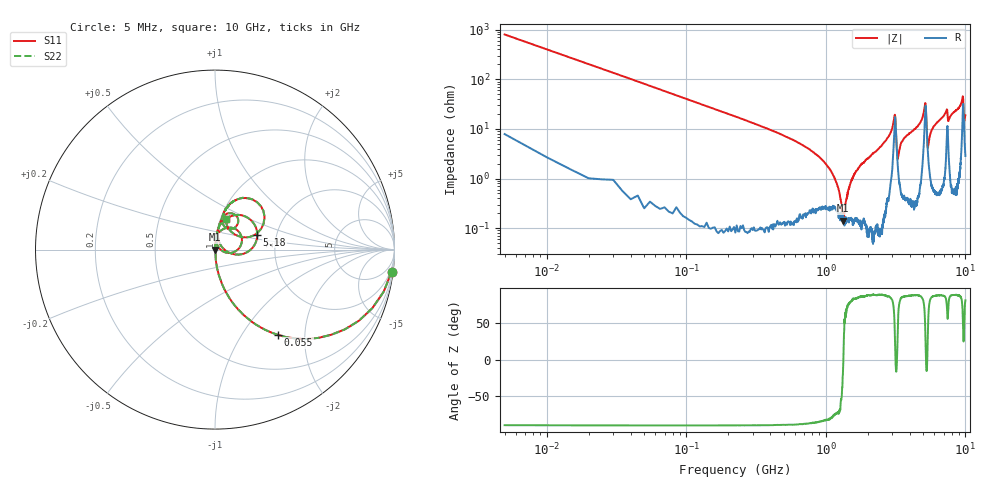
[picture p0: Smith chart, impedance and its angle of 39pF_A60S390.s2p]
! Amotech Co.,Ltd.
! http://www.amotech.co.kr/
! Part Number: A60S390
! These Parameters are Measured in Series Mode Connection
! Operation Temp=25[degC], DC Bias Voltage=0[V]
! Freq. Start=5[MHz] Stop=10[GHz], 2000[Steps]
! Date: Monday, July 13, 2020, 01:42:09
# GHZ S RI R 50.000000
!Freq.(Hz) S11(Real) S11(Imag) S21(Real) S21(Imag) S12(Real) S12(Imag) S22(Real) S22(Imag)
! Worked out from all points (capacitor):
!   2000 points, 5 MHz to 10 GHz, reference 50 ohm
!   read as one part in series: C = 39.1 pF near 55 MHz
!   lowest |Z| = 142 mohm at 1.335 GHz (marker M1)
!   series resonance near 1.336 GHz, so ESL is about 360 pH
!   S11 on the Smith chart (normalised r, x): 5 MHz: 1, -16; 55 MHz: 1.01, -1.47; 5.18 GHz: 1.58, +0.28; 10 GHz: 1.06, +0.37
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0.005  0.9834 -0.1229  0.0166 0.1229  0.0166 0.1229  0.9834 -0.1229
0.055  0.3526 -0.4755  0.6474 0.4755  0.6474 0.4755  0.3526 -0.4755
0.11  0.1204 -0.3236  0.8796 0.3236  0.8796 0.3236  0.1204 -0.3236
0.215  0.0344 -0.1797  0.9656 0.1797  0.9656 0.1797  0.0344 -0.1797
1.065  0.00248 -0.0153  0.9975 0.0153  0.9975 0.0153  0.00248 -0.0153
1.335  0.00142 -6.45e-05  0.9986 6.45e-05  0.9986 6.45e-05  0.00142 -6.45e-05
1.5  0.00163 0.00795  0.9984 -0.00795  0.9984 -0.00795  0.00163 0.00795
1.675  0.0018 0.0146  0.9982 -0.0146  0.9982 -0.0146  0.0018 0.0146
3.1  0.1076 0.1175  0.8924 -0.1175  0.8924 -0.1175  0.1076 0.1175
3.15  0.1381 0.0129  0.8619 -0.0129  0.8619 -0.0129  0.1381 0.0129
3.255  0.0238 0.00785  0.9762 -0.00785  0.9762 -0.00785  0.0238 0.00785
3.34  0.0108 0.032  0.9892 -0.032  0.9892 -0.032  0.0108 0.032
3.63  0.00833 0.0639  0.9917 -0.0639  0.9917 -0.0639  0.00833 0.0639
5.005  0.0677 0.1775  0.9323 -0.1775  0.9323 -0.1775  0.0677 0.1775
5.18  0.2354 0.0833  0.7646 -0.0833  0.7646 -0.0833  0.2354 0.0833
5.39  0.0315 0.0251  0.9685 -0.0251  0.9685 -0.0251  0.0315 0.0251
5.74  0.0158 0.0934  0.9842 -0.0934  0.9842 -0.0934  0.0158 0.0934
6.67  0.0296 0.1531  0.9704 -0.1531  0.9704 -0.1531  0.0296 0.1531
8.335  0.0512 0.2081  0.9488 -0.2081  0.9488 -0.2081  0.0512 0.2081
9.545  0.2345 0.263  0.7655 -0.263  0.7655 -0.263  0.2345 0.263
9.795  0.1005 0.0912  0.8995 -0.0912  0.8995 -0.0912  0.1005 0.0912
10  0.0586 0.1705  0.9414 -0.1705  0.9414 -0.1705  0.0586 0.1705
